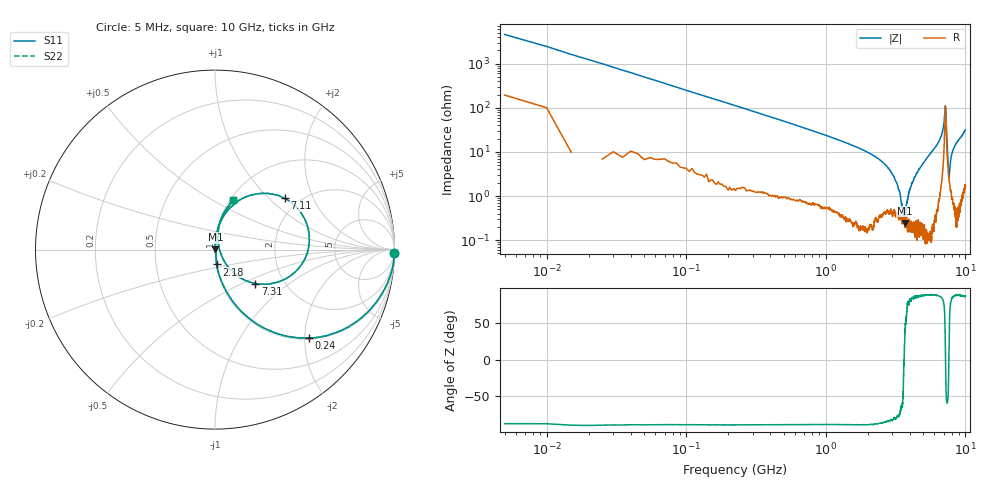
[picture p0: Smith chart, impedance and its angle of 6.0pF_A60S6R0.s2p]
! Amotech Co.,Ltd.
! http://www.amotech.co.kr/
! Part Number: A60S6R0
! These Parameters are Measured in Series Mode Connection
! Operation Temp=25[degC], DC Bias Voltage=0[V]
! Freq. Start=5[MHz] Stop=10[GHz], 2000[Steps]
! Date: Monday, July 13, 2020, 01:31:02
# GHZ S RI R 50.000000
!Freq.(Hz) S11(Real) S11(Imag) S21(Real) S21(Imag) S12(Real) S12(Imag) S22(Real) S22(Imag)
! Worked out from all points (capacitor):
!   2000 points, 5 MHz to 10 GHz, reference 50 ohm
!   read as one part in series: C = 6.36 pF near 55 MHz
!   lowest |Z| = 243 mohm at 3.665 GHz (marker M1)
!   series resonance near 3.636 GHz, so ESL is about 300 pH
!   S11 on the Smith chart (normalised r, x): 5 MHz: 5, -92; 240 MHz: 1.03, -2.09; 2.18 GHz: 1.00, -0.17; 7.11 GHz: 1.68, +1.25; 7.31 GHz: 1.43, -0.59; 10 GHz: 1.03, +0.63
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0.005  0.9986 -0.0217  0.00139 0.0217  0.00139 0.0217  0.9986 -0.0217
0.09  0.8814 -0.3152  0.1186 0.3152  0.1186 0.3152  0.8814 -0.3152
0.24  0.5227 -0.4922  0.4773 0.4922  0.4773 0.4922  0.5227 -0.4922
0.415  0.2703 -0.4355  0.7297 0.4355  0.7297 0.4355  0.2703 -0.4355
0.655  0.1294 -0.3253  0.8706 0.3253  0.8706 0.3253  0.1294 -0.3253
1.675  0.0182 -0.1246  0.9818 0.1246  0.9818 0.1246  0.0182 -0.1246
2.18  0.00865 -0.0827  0.9914 0.0827  0.9914 0.0827  0.00865 -0.0827
2.895  0.00587 -0.0369  0.9941 0.0369  0.9941 0.0369  0.00587 -0.0369
3.34  0.00344 -0.0129  0.9966 0.0129  0.9966 0.0129  0.00344 -0.0129
3.665  0.00227 0.000863  0.9977 -0.000863  0.9977 -0.000863  0.00227 0.000863
3.825  0.00246 0.0074  0.9975 -0.0074  0.9975 -0.0074  0.00246 0.0074
4.125  0.00213 0.0187  0.9979 -0.0187  0.9979 -0.0187  0.00213 0.0187
5.005  0.00428 0.0564  0.9957 -0.0564  0.9957 -0.0564  0.00428 0.0564
6.67  0.0568 0.1995  0.9432 -0.1995  0.9432 -0.1995  0.0568 0.1995
6.95  0.1483 0.2832  0.8517 -0.2832  0.8517 -0.2832  0.1483 0.2832
7.11  0.3878 0.2857  0.6122 -0.2857  0.6122 -0.2857  0.3878 0.2857
7.2  0.5198 0.00243  0.4802 -0.00243  0.4802 -0.00243  0.5198 0.00243
7.31  0.2239 -0.189  0.7761 0.189  0.7761 0.189  0.2239 -0.189
7.625  0.0241 0.00506  0.9759 -0.00506  0.9759 -0.00506  0.0241 0.00506
7.92  0.0171 0.0759  0.9829 -0.0759  0.9829 -0.0759  0.0171 0.0759
8.335  0.0214 0.127  0.9786 -0.127  0.9786 -0.127  0.0214 0.127
10  0.1027 0.2785  0.8973 -0.2785  0.8973 -0.2785  0.1027 0.2785
